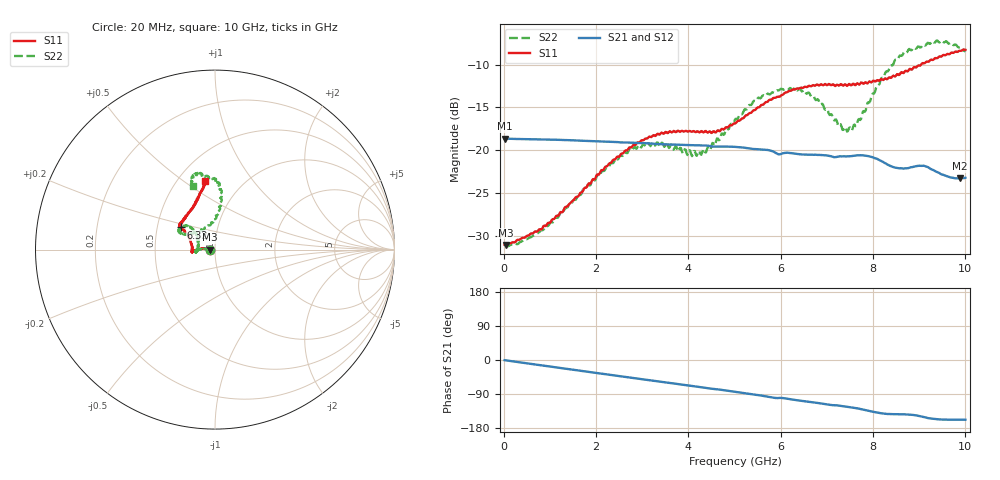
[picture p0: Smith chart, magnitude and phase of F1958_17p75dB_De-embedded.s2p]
! Integrated Device Technology
! Corporate Headquarters
! 6024 Silver Creek Valley Road
! San Jose, CA 95138  USA
! Phone:  1-408-284-8200
! Toll Free:  1-800-223-1366
! Webpage:  http://www.idt.com/
! Timing and RF Division
! 515 Groton Road, Suite 102
! Westford, MA 01886-6024
! Device:  F1958
! Description: 7-bit 0.25 dB Digital Step Attenuator
! Frequency:  0.001 -  6.000 GHz
! Package:  4x4 mm Thin QFN Plastic Package: 24 pin
! Ports:  2 RF, 12 DC
!  Pin  1  = D0
!  Pin  2  = VDD
!  Pin  3  = VMODE
!  Pin  4  = GND
!  Pin  5  = RF1  =  Port 1
!  Pin  6  = GND
!  Pin  7  = GND
!  Pin  8  = GND
!  Pin  9  = GND
!  Pin 10  = GND
!  Pin 11  = GND
!  Pin 12  = GND
!  Pin 13  = GND
!  Pin 14  = RF2  =  Port 2
!  Pin 15  = GND
!  Pin 16  = LE
!  Pin 17  = CLK
!  Pin 18  = DATA
!  Pin 19  = D6
!  Pin 20  = D5
!  Pin 21  = D4
!  Pin 22  = D3
!  Pin 23  = D2
!  Pin 24  = D1
! State:  71
! Atten State:  17.75 dB
! Voltage:  +3.30 Volts
! Current:  0.258 mA
! Data:  The device was measured on a F1958 evaluation board which has
!  individual transmission lines to the RF pins.  Data was collected
!  using a calibrated network analyzer.  The evaluation board was
!  de-embedded using Automatic Fixture Removal (AFR).
!  The reference plane is the edge of the package pin.
! Misc:
!  Action Tracker AT0419
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# GHz S dB R 50
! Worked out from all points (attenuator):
!   500 points, 20 MHz to 10 GHz, reference 50 ohm
!   highest |S21| = -18.64 dB at 20 MHz (marker M1); lowest = -23.3 dB at 9.88 GHz (marker M2)
!   lowest |S11| = -31.1 dB at 40 MHz (marker M3), VSWR 1.06, Z = 47.3 - j0.068 ohm
!   |S11| at or under -10 dB: start of sweep to 9.041 GHz
!   |S22| runs from -31.2 to -7.2 dB; largest |S21 - S12| = 0.00037
!   S11 on the Smith chart (normalised r, x): 20 MHz: 0.95, -0.00; 6.32 GHz: 0.66, +0.17; 10 GHz: 0.68, +0.61
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0.02  -31.05 -178.4  -18.64 -0.5  -18.64 -0.4  -31.05 -178.8
0.04  -31.08 -178.5  -18.65 -0.8  -18.64 -0.8  -31.02 -178.1
0.32  -30.46 177.0  -18.69 -5.7  -18.68 -5.6  -30.91 177.0
0.84  -29.09 174.7  -18.74 -14.5  -18.73 -14.5  -29.35 176.5
1.7  -24.90 175.5  -18.89 -29.0  -18.88 -29.0  -24.83 175.3
2.62  -20.11 -180.0  -19.09 -44.4  -19.07 -44.4  -20.22 -178.5
3.36  -18.15 -174.2  -19.28 -56.8  -19.28 -56.9  -19.38 -171.3
4.24  -17.92 -178.8  -19.43 -71.1  -19.44 -71.2  -20.12 166.9
4.5  -17.98 175.4  -19.56 -75.8  -19.57 -75.8  -19.49 151.5
5.02  -16.85 161.0  -19.61 -84.1  -19.62 -84.1  -16.33 138.5
5.56  -14.82 150.4  -19.90 -93.5  -19.91 -93.5  -13.93 139.6
5.98  -13.72 148.1  -20.48 -100.0  -20.49 -100.0  -12.92 146.2
6.32  -12.87 147.1  -20.40 -105.7  -20.41 -105.7  -12.77 152.8
6.68  -12.44 145.5  -20.52 -111.2  -20.54 -111.1  -13.67 153.4
7.3  -12.27 139.4  -20.71 -121.1  -20.72 -121.0  -16.97 132.8
7.5  -12.30 136.6  -20.70 -124.4  -20.71 -124.3  -17.34 114.8
7.7  -12.34 132.6  -20.58 -128.6  -20.59 -128.6  -16.35 98.3
8.34  -11.50 117.6  -21.74 -142.6  -21.75 -142.8  -10.62 82.8
8.7  -10.72 111.1  -22.12 -143.5  -22.11 -143.4  -8.53 88.2
9.26  -9.41 103.2  -22.22 -154.4  -22.21 -154.6  -7.36 99.7
9.88  -8.36 98.6  -23.30 -157.4  -23.33 -157.3  -7.95 108.5
10  -8.27 98.2  -23.21 -157.7  -23.25 -157.7  -8.47 109.1
